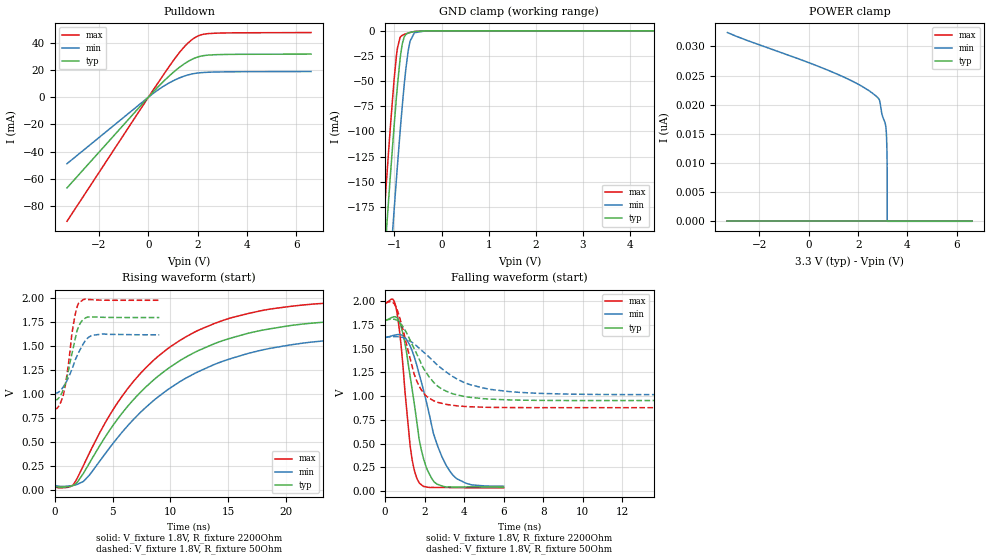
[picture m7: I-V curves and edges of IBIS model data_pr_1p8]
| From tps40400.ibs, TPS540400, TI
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|   data_pr_1p8 Model
[Model]   data_pr_1p8
Model_type   I/O_open_drain
Polarity   Inverting
Vinl = 0.8
Vinh = 2.1
Vmeas = 1.65
Vref = 3.3
Cref = 2pF
Rref = 2200
|   typ   min   max
|   (nom PVT)   (fast PVT)   (slow PVT)
 C_comp   1.617e-12   1.585e-12   1.729e-12
| Where nom  PVT is Nominal Process, 3.3V, 25C
|   Fast PVT is Strong Process,  3.4V, -40C
|   Slow PVT is Weak Process,   3.2V, 125C
[Voltage Range]   3.3   3.2   3.4
|Junction Temperature
[Temperature Range]   25   125   -40
[Pullup Reference]   3.3   3.2   3.4
[Pulldown Reference]   0   0   0
[Power Clamp Reference]   3.3   3.2   3.4
[GND Clamp Reference]   0   0   0
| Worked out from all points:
|   slope of the pulldown table from 0 to 0.495 V, typ, clamps not added: 52.4 ohm
|   GND clamp passes 1 mA (typ) near -0.60 V on its own axis
|   falling waveform, V_fixture 1.8V, R_fixture 2200Ohm: 20-80 % time 789ps typ, 1.24ns min, 524ps max; typ from 1.8 V to 0.04 V
|   rising waveform, V_fixture 1.8V, R_fixture 2200Ohm: 20-80 % time 8.77ns typ, 9.46ns min, 8.09ns max; typ from 0.04 V to 1.8 V
|   falling waveform, V_fixture 1.8V, R_fixture 50Ohm: 20-80 % time 1.42ns typ, 2.34ns min, 955ps max; typ from 1.8 V to 0.945 V
|   rising waveform, V_fixture 1.8V, R_fixture 50Ohm: 20-80 % time 935ps typ, 1.32ns min, 766ps max; typ from 0.942 V to 1.8 V
[Pulldown]
|   Voltage   I(typ)   I(min)   I(max)
-3.3V     -66.53mA   -48.77mA   -91.01mA
257.4mV   5.028mA    3.596mA    6.933mA
814mV     15.05mA    10.18mA    21.76mA
1.253V    21.83mA    14.09mA    32.62mA
1.48V     24.77mA    15.62mA    37.4mA
1.756V    27.65mA    16.98mA    42.03mA
2.046V    29.71mA    17.82mA    45.17mA
2.439V    30.88mA    18.3mA     46.63mA
6.597V    31.61mA    18.84mA    47.39mA
[GND Clamp]
|   Voltage   I(typ)   I(min)   I(max)
-3.3V     -1.648A    -1.717A    -1.608A
-1.27V    -266.7mA   -355.3mA   -219.2mA
-1.165V   -195.4mA   -282.8mA   -146.8mA
-1.089V   -145.8mA   -231.9mA   -97.3mA
-1.009V   -95.8mA    -179.6mA   -49.55mA
-937mV    -54.97mA   -134.6mA   -17.46mA
-865.6mV  -22.65mA   -92.4mA    -5.675mA
-792mV    -6.034mA   -53.46mA   -3.563mA
-665mV    -1.602mA   -9.956mA   -1.625mA
-573.6mV  -736.5uA   -1.829mA   -633uA
-330.4mV  -7.166uA   -42.24uA   -2.454uA
6.597V    0A         0A         0A
[POWER Clamp]
|   Voltage   I(typ)   I(min)   I(max)
-3.3V     0A         32.36nA    0A
1.253V    0A         25.04nA    0A
2.153V    0A         23.15nA    0A
2.835V    0A         21.01nA    0A
2.886V    0A         20.41nA    0A
2.976V    0A         18.19nA    0A
3.103V    0A         16.67nA    0A
3.138V    0A         15.44nA    0A
3.158V    0A         13.55nA    0A
3.175V    0A         10.01nA    0A
3.177V    0A         0A         0A
6.597V    0A         0A         0A
[Ramp]
R_load = 2200
|   typ   min   max
dV/dt_r   1.05595/8.77102e-09   0.94238/9.44697e-09   1.16851/8.09452e-09
dV/dt_f   1.05597/7.87193e-10   0.942418/1.24098e-09   1.16853/5.20844e-10
[Falling Waveform]
V_fixture = 1.8V
V_fixture_min = 1.62V
V_fixture_max = 1.98V
R_fixture = 2200Ohm
|   Time   V(typ)   V(min)   V(max)
0s        1.8V       1.62V      1.98V
390ps     1.832V     1.638V     2.022V
595ps     1.828V     1.647V     1.893V
920ps     1.647V     1.635V     1.291V
1.275ns   1.205V     1.527V     471.4mV
1.73ns    542.1mV    1.231V     85.11mV
2.435ns   109.6mV    618.5mV    37.21mV
3.285ns   43.35mV    207.5mV    35.67mV
4.1ns     42.41mV    80.72mV    33.9mV
6ns       40.06mV    49.25mV    32.46mV
[Rising Waveform]
V_fixture = 1.8V
V_fixture_min = 1.62V
V_fixture_max = 1.98V
R_fixture = 2200Ohm
|   Time   V(typ)   V(min)   V(max)
0s        40.05mV    49.25mV    32.46mV
1.62ns    51.1mV     49.46mV    60.05mV
2.99ns    280.3mV    155.4mV    385.4mV
5.07ns    680.6mV    491.8mV    843.8mV
8.52ns    1.146V     931mV      1.351V
12.27ns   1.446V     1.226V     1.658V
16.74ns   1.636V     1.426V     1.842V
22.5ns    1.744V     1.548V     1.942V
29.78ns   1.788V     1.601V     1.975V
70ns      1.8V       1.62V      1.98V
[Falling Waveform]
V_fixture = 1.8V
V_fixture_min = 1.62V
V_fixture_max = 1.98V
R_fixture = 50Ohm
|   Time   V(typ)   V(min)   V(max)
0s        1.8V       1.62V      1.98V
370ps     1.811V     1.627V     1.992V
570ps     1.804V     1.627V     1.933V
960ps     1.713V     1.614V     1.658V
1.47ns    1.504V     1.551V     1.236V
2.045ns   1.261V     1.447V     1.009V
2.875ns   1.074V     1.289V     923.9mV
4.98ns    972.6mV    1.085V     882.8mV
14.1ns    953.5mV    1.015V     877.5mV
200ns     945.5mV    1.015V     855.5mV
[Rising Waveform]
V_fixture = 1.8V
V_fixture_min = 1.62V
V_fixture_max = 1.98V
R_fixture = 50Ohm
|   Time   V(typ)   V(min)   V(max)
0s        942.2mV    1.014V     847.8mV
410ps     972.1mV    1.029V     889.4mV
800ps     1.068V     1.088V     1.023V
1.105ns   1.201V     1.154V     1.247V
1.6ns     1.485V     1.298V     1.719V
1.875ns   1.637V     1.386V     1.888V
2.14ns    1.726V     1.453V     1.963V
2.68ns    1.797V     1.565V     1.992V
3.185ns   1.804V     1.612V     1.987V
9.045ns   1.8V       1.62V      1.98V
